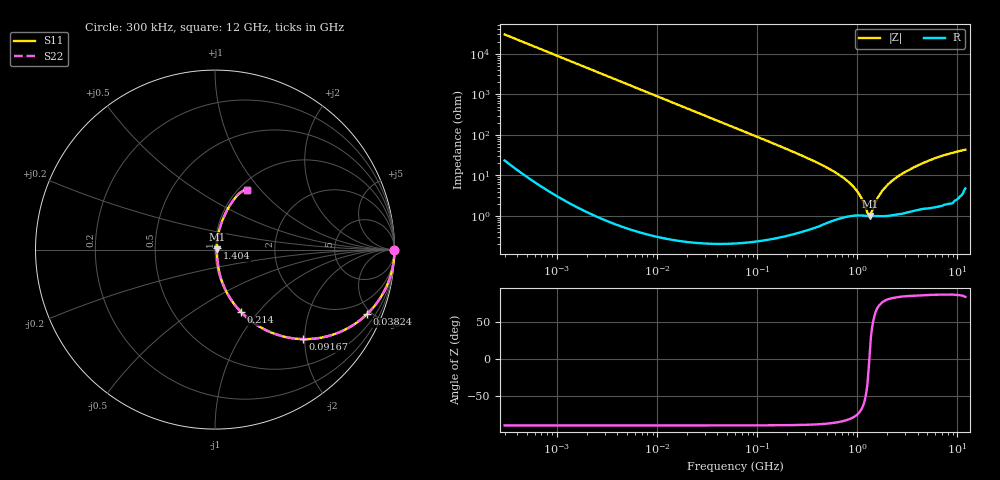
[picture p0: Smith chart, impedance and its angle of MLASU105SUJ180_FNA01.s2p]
! MLASU105SUJ180_FNA01  S-PARAMETER MODEL  ( General Type )
! Model Generated by TAIYO YUDEN Corporation (http://www.ty-top.com)
! Version 2.0
! TAIYO YUDEN Control No. 120810
! Copyright(c) 2012 TAIYO YUDEN CO.,LTD. All Rights Reserved.
! Product Description (link to TY-COMPAS)
! https://ds.yuden.co.jp/TYCOMPAS/or/detail?pn=MLASU105SUJ180JFNA01&u=M
! Products Name : Multilayer Ceramic Capacitors
! Characteristics :
!  Capacitance : 18 pF , Rated Voltage : 50V , TCC : UJ / U2J
!  Case Size : 1.0 x 0.5 / 0.039 x 0.02 [mm/inch] , Thickness : 0.5 / 0.02 [mm/inch]
!  (Conditions: Temperature = 25 degC , DC Bias Current/Voltage = 0A / 0V)
! External Node Assignments :
!  1  o---| |---o  2
! GND o---------o GND
! Frequency Range : 0.3MHz  -  12000MHz  [ 401 STEP ]
# MHz S RI R 50
! Freq[MHz].  S11 Real  S11 Imag  S21 Real  S21 Imag  S12 Real  S12 Imag  S22 Real  S22 Imag
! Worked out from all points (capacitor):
!   401 points, 300 kHz to 12 GHz, reference 50 ohm
!   read as one part in series: C = 17.7 pF near 316.3 kHz
!   lowest |Z| = 996 mohm at 1.331 GHz (marker M1)
!   series resonance near 1.318 GHz, so ESL is about 820 pH
!   S11 on the Smith chart (normalised r, x): 300 kHz: open; 38.24 MHz: 1.00, -4.70; 91.67 MHz: 1.00, -1.95; 214 MHz: 1.01, -0.82; 1.404 GHz: 1.02, +0.02; 12 GHz: 1.10, +0.85
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0.3  1 -0.00333  1.37e-05 0.00333  1.37e-05 0.00333  1 -0.00333
1.769972  0.9996 -0.0197  0.000392 0.0197  0.000392 0.0197  0.9996 -0.0197
10.44266  0.9867 -0.1145  0.0133 0.1145  0.0133 0.1145  0.9867 -0.1145
21.92581  0.9438 -0.23  0.0562 0.23  0.0562 0.23  0.9438 -0.23
38.24403  0.8466 -0.36  0.1534 0.36  0.1534 0.36  0.8466 -0.36
60  0.6911 -0.4613  0.3089 0.4613  0.3089 0.4613  0.6911 -0.4613
91.67136  0.4883 -0.4987  0.5117 0.4987  0.5117 0.4987  0.4883 -0.4987
213.9924  0.1457 -0.3487  0.8543 0.3487  0.8543 0.3487  0.1457 -0.3487
353.9943  0.0569 -0.2216  0.9431 0.2216  0.9431 0.2216  0.0569 -0.2216
601.3112  0.0215 -0.1153  0.9785 0.1153  0.9785 0.1153  0.0215 -0.1153
848.5281  0.0136 -0.0611  0.9864 0.0611  0.9864 0.0611  0.0136 -0.0611
1021.415  0.0114 -0.035  0.9886 0.035  0.9886 0.035  0.0114 -0.035
1135.593  0.0106 -0.0206  0.9894 0.0206  0.9894 0.0206  0.0106 -0.0206
1262.535  0.00986 -0.00645  0.9901 0.00645  0.9901 0.00645  0.00986 -0.00645
1331.232  0.00976 0.00144  0.9902 -0.00144  0.9902 -0.00144  0.00976 0.00144
1403.667  0.00989 0.00888  0.9901 -0.00888  0.9901 -0.00888  0.00989 0.00888
1689.663  0.0108 0.0322  0.9892 -0.0322  0.9892 -0.0322  0.0108 0.0322
2088.533  0.0139 0.0617  0.9861 -0.0617  0.9861 -0.0617  0.0139 0.0617
2870.14  0.0236 0.1095  0.9764 -0.1095  0.9764 -0.1095  0.0236 0.1095
4747.894  0.056 0.197  0.944 -0.197  0.944 -0.197  0.056 0.197
7448.838  0.1052 0.2784  0.8948 -0.2784  0.8948 -0.2784  0.1052 0.2784
12000  0.1808 0.3329  0.8192 -0.3329  0.8192 -0.3329  0.1808 0.3329
